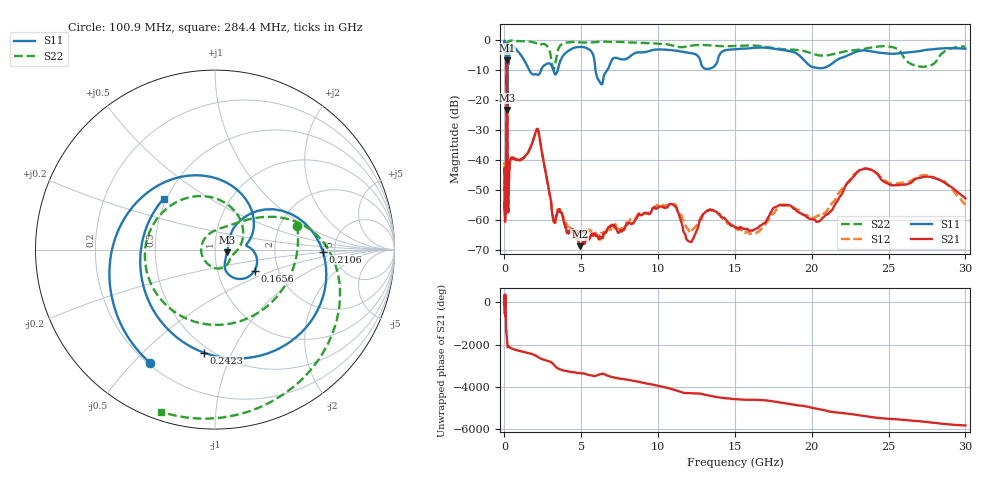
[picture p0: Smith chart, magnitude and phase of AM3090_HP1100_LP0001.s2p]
! Date/Time: Thu, Feb 28, 2019 2:06 PM
! Network Analyzer: Agilent Technologies E8364B Rev: A.07.50.67
! Sweep from 0.010 to 30.000 GHz, 1601 Points, Sweep Type: LOG
! Power Supply: 5.022 V, 0.002 A
# Hz S DB R 50
!freq MagS11 AngS11 MagS21 AngS21 MagS12 AngS12 MagS22 AngS22
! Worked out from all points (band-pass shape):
!   1601 points, 10 MHz to 30 GHz, reference 50 ohm
!   highest |S21| = -6.76 dB at 158.3 MHz (marker M1); lowest = -68.6 dB at 4.903 GHz (marker M2)
!   |S21| within 3 dB of the highest: 139.8 MHz to 182.6 MHz (42.86 MHz wide, 26.6 % of centre)
!   lowest |S11| = -23.3 dB at 186.8 MHz (marker M3), VSWR 1.15, Z = 57.1 - j1.73 ohm
!   |S11| at or under -10 dB: 1.61 GHz to 2.387 GHz (777.2 MHz wide, 38.9 % of centre); 3.181 GHz to 3.465 GHz (283.8 MHz wide, 8.54 % of centre); 5.926 GHz to 6.694 GHz (768.5 MHz wide, 12.2 % of centre)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
!   |S22| runs from -22.2 to -0.1 dB; largest |S21 - S12| = 0.013
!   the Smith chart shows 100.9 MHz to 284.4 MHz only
!   S11 on the Smith chart (normalised r, x): 100.9 MHz: 0.21, -0.56; 165.6 MHz: 1.51, -0.38; 210.6 MHz: 4.01, -0.14; 242.3 MHz: 0.46, -0.79; 284.4 MHz: 0.48, +0.33
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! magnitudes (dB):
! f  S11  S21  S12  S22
! 10 MHz  -0.3  -44.3  -41.0  -0.5
! 38.04 MHz  -0.4  -56.5  -58.5  -1.2
! 100.9 MHz  -2.8  -53.5  -51.9  -6.4
! 144.7 MHz  -14.6  -7.9  -7.9  -19.1
! 158.3 MHz  -12.8  -6.8  -6.7  -19.2
! 165.6 MHz  -12.1  -7.0  -6.9  -20.7
! 186.8 MHz  -23.3  -11.9  -11.9  -14.4
! 210.6 MHz  -4.4  -50.4  -50.0  -2.4
! 242.3 MHz  -4.8  -56.5  -54.9  -0.7
! 284.4 MHz  -7.9  -47.5  -46.8  -0.4
! 550.5 MHz  -2.1  -39.4  -39.3  -0.2
! 2.084 GHz  -11.5  -29.9  -29.9  -1.2
! 3.22 GHz  -10.7  -60.4  -60.4  -9.6
! 4.903 GHz  -2.3  -68.6  -63.8  -0.8
! 6.234 GHz  -14.2  -65.8  -66.5  -0.6
! 7.926 GHz  -6.3  -61.7  -60.8  -0.8
! 10.7 GHz  -3.3  -54.8  -55.0  -1.5
! 12.07 GHz  -4.3  -67.2  -64.0  -2.0
! 16.21 GHz  -2.6  -63.2  -64.5  -1.8
! 20.61 GHz  -9.4  -59.8  -57.7  -5.2
! 23.48 GHz  -3.5  -42.8  -42.8  -2.9
! 30 GHz  -2.9  -52.7  -54.8  -2.1
